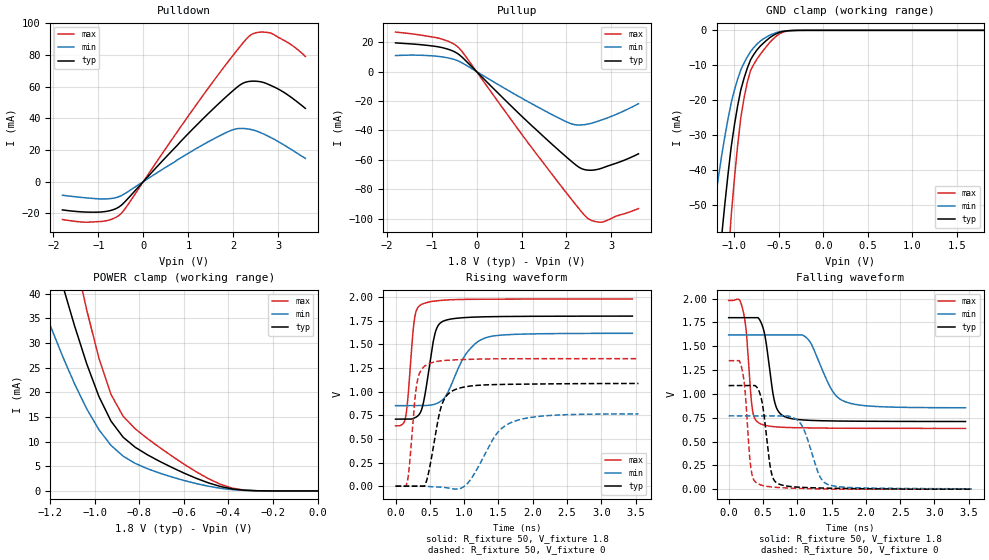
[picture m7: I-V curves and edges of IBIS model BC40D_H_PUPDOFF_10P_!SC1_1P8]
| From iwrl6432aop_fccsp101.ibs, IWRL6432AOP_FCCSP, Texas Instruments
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|   Model Cell BC40D_H_PUPDOFF_10P_!SC1_1P8
|BC40D_H_PUPDOFF_10P_!SC1_1P8
[Model]   BC40D_H_PUPDOFF_10P_!SC1_1P8
Model_type   I/O
Polarity   Non-Inverting
Enable   Active-Low
Vinl =  0.63
Vinh =  1.17
Cref =  15pF
Rref =  100.0000M
Vref =  0V
Vmeas =  0.9
C_comp   2.389419p   2.292106p   2.408415p
|[Input load] weak_pupdoff
|[Output drive] fast
|[supplytol] 10
|[temp] ind
[Model Spec]
Vinl   0.63   0.567   0.693
Vinh   1.17   1.053   1.287
[Temperature Range]   25   125   -40
[Voltage Range]   1.8   1.62   1.98
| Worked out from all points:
|   slope of the pulldown table from 0 to 0.27 V, typ, clamps not added: 32.2 ohm
|   slope of the pullup table from 0 to 0.27 V, typ, clamps not added: 32.5 ohm
|   GND clamp passes 1 mA (typ) near -0.53 V on its own axis
|   POWER clamp passes 1 mA (typ) near -0.44 V on its own axis
|   rising waveform, R_fixture 50, V_fixture 1.8: 20-80 % time 145ps typ, 331ps min, 89ps max; typ from 0.709 V to 1.8 V
|   rising waveform, R_fixture 50, V_fixture 0: 20-80 % time 176ps typ, 382ps min, 101ps max; typ from 0 V to 1.09 V
|   falling waveform, R_fixture 50, V_fixture 1.8: 20-80 % time 130ps typ, 293ps min, 86.1ps max; typ from 1.8 V to 0.71 V
|   falling waveform, R_fixture 50, V_fixture 0: 20-80 % time 113ps typ, 213ps min, 82.8ps max; typ from 1.09 V to 0 V
| Nom Voltages:
|   VDD=1.1001, VDDS=1.8, VDDS18=1.8, ESD_BIASFET=0, VSS=0, VSSS=0
| Min Voltages:
|   VDD=0.99, VDDS=1.62, VDDS18=1.62, ESD_BIASFET=0, VSS=0, VSSS=0
| Max Voltages:
|   VDD=1.21, VDDS=1.98, VDDS18=1.98, ESD_BIASFET=0, VSS=0, VSSS=0
[POWER_clamp]
|   voltage   I(typ)   I(min)   I(max)
-1.8V     158.8mA    112.5mA    219.7mA
-1.255V   59.93mA    40mA       84.85mA
-1.127V   39.08mA    25.51mA    55.74mA
-1.055V   28.36mA    18.34mA    40.4mA
-981.8mV  19.18mA    12.43mA    26.97mA
-927.3mV  14.16mA    9.242mA    19.58mA
-872.7mV  10.89mA    7.052mA    15.14mA
-818.2mV  8.843mA    5.581mA    12.58mA
-600mV    3.63mA     2.129mA    5.448mA
-436.4mV  903.9uA    539.1uA    1.358mA
-327.3mV  138.2uA    94.86uA    160.4uA
0V        19.3nA     120.3nA    352.8nA
[Pulldown]
|   voltage   I(typ)   I(min)   I(max)
-1.8V     -17.92mA   -8.674mA   -24.03mA
-927.3mV  -19.22mA   -10.99mA   -25.2mA
-654.5mV  -17.65mA   -10.46mA   -23.22mA
-490.9mV  -14.97mA   -8.904mA   -20.12mA
872.7mV   26.63mA    15.72mA    36.29mA
1.691V    49.7mA     28.87mA    68.59mA
2.127V    60.63mA    33.53mA    84.59mA
2.4V      63.43mA    32.84mA    92.9mA
2.618V    62.99mA    30.74mA    94.47mA
2.836V    60.69mA    27.76mA    93.76mA
3.273V    53.49mA    20.53mA    86.73mA
3.6V      46.26mA    14.64mA    79.11mA
[Pullup]
|   voltage   I(typ)   I(min)   I(max)
-1.8V     19.47mA    10.86mA    26.81mA
-818.2mV  16.61mA    10.18mA    22.5mA
-545.5mV  14.21mA    8.665mA    19.39mA
-381.8mV  11.35mA    6.855mA    15.77mA
1.036V    -31.31mA   -18.66mA   -43.94mA
1.909V    -55.72mA   -32.86mA   -78.99mA
2.182V    -62.87mA   -36.1mA    -89.59mA
2.345V    -66.12mA   -36.26mA   -95.76mA
2.455V    -66.95mA   -35.82mA   -99.33mA
2.618V    -66.9mA    -34.58mA   -101.8mA
2.782V    -65.72mA   -32.89mA   -102.4mA
3.6V      -55.92mA   -21.86mA   -93.15mA
[GND_clamp]
|   voltage   I(typ)   I(min)   I(max)
-1.8V     -270.2mA   -170.2mA   -430.1mA
-1.255V   -91.66mA   -55.91mA   -148.4mA
-1.145V   -59.91mA   -36.44mA   -97.09mA
-1.109V   -50.48mA   -30.83mA   -81.55mA
-1.073V   -41.73mA   -25.65mA   -67.05mA
-1.036V   -33.66mA   -20.92mA   -53.59mA
-927.3mV  -17.07mA   -11.35mA   -25.04mA
-854.5mV  -10.86mA   -7.616mA   -14.91mA
-781.8mV  -6.919mA   -4.945mA   -9.771mA
-636.4mV  -2.823mA   -1.868mA   -4.529mA
-381.8mV  -84.73uA   -78.7uA    -126.1uA
1.8V      19.3nA     3.129uA    310.3nA
[Ramp]
| variable   typ   min   max
dV/dt_f 0.66537664/0.13285487n 0.47054269/0.29993714n 0.81466395/87.718121p
dV/dt_r 0.66473017/0.17862173n 0.48133529/0.39881724n 0.81910029/0.10167218n
R_load = 50
[Rising Waveform]
R_fixture = 50
V_fixture = 1.8
V_fixture_min = 1.62
V_fixture_max = 1.98
|   time   V(typ)   V(min)   V(max)
0s        709.3mV    852.1mV    638.7mV
143.5ps   709.3mV    852.1mV    719.5mV
180.9ps   709.3mV    852.1mV    942.5mV
270.5ps   720.3mV    852.1mV    1.741V
373.4ps   797.8mV    852.1mV    1.921V
571.3ps   1.605V     867.4mV    1.959V
699.1ps   1.747V     923.9mV    1.968V
1.017ns   1.784V     1.388V     1.977V
1.315ns   1.793V     1.571V     1.979V
3.453ns   1.8V       1.618V     1.98V
[Rising Waveform]
R_fixture = 50
V_fixture = 0
V_fixture_min = 0
V_fixture_max = 0
|   time   V(typ)   V(min)   V(max)
0s        0V         0V         0V
168.3ps   0V         0V         39.19mV
311.9ps   0V         0V         1.091V
464.8ps   90.04mV    -2.657mV   1.289V
661.8ps   832.6mV    -10.42mV   1.326V
859.7ps   1.019V     -30.72mV   1.336V
1.065ns   1.057V     42.97mV    1.342V
1.47ns    1.075V     550.3mV    1.348V
1.69ns    1.078V     675mV      1.349V
3.542ns   1.087V     765.1mV    1.35V
[Falling Waveform]
R_fixture = 50
V_fixture = 1.8
V_fixture_min = 1.62
V_fixture_max = 1.98
|   time   V(typ)   V(min)   V(max)
0s        1.8V       1.619V     1.981V
201.7ps   1.8V       1.619V     1.898V
255.7ps   1.8V       1.619V     1.659V
345.5ps   1.8V       1.619V     838.7mV
451.6ps   1.778V     1.619V     690.5mV
673.3ps   907.3mV    1.619V     654.8mV
807.1ps   764.8mV    1.619V     648.7mV
1.149ns   723.5mV    1.58V      643.6mV
1.693ns   714.4mV    919.6mV    639.4mV
3.453ns   710.3mV    854.5mV    638mV
[Falling Waveform]
R_fixture = 50
V_fixture = 0
V_fixture_min = 0
V_fixture_max = 0
|   time   V(typ)   V(min)   V(max)
0s        1.088V     769.7mV    1.349V
186.8ps   1.088V     769.7mV    1.284V
238.3ps   1.088V     769.7mV    1.038V
324.1ps   1.088V     769.7mV    220.2mV
424.5ps   1.056V     769.7mV    57.79mV
618.8ps   186mV      769.7mV    23.68mV
725.8ps   55.9mV     769.7mV    16.99mV
1.045ns   19.62mV    691.6mV    7.785mV
1.455ns   10.34mV    47.08mV    2.036mV
3.542ns   0V         3.732mV    0V
